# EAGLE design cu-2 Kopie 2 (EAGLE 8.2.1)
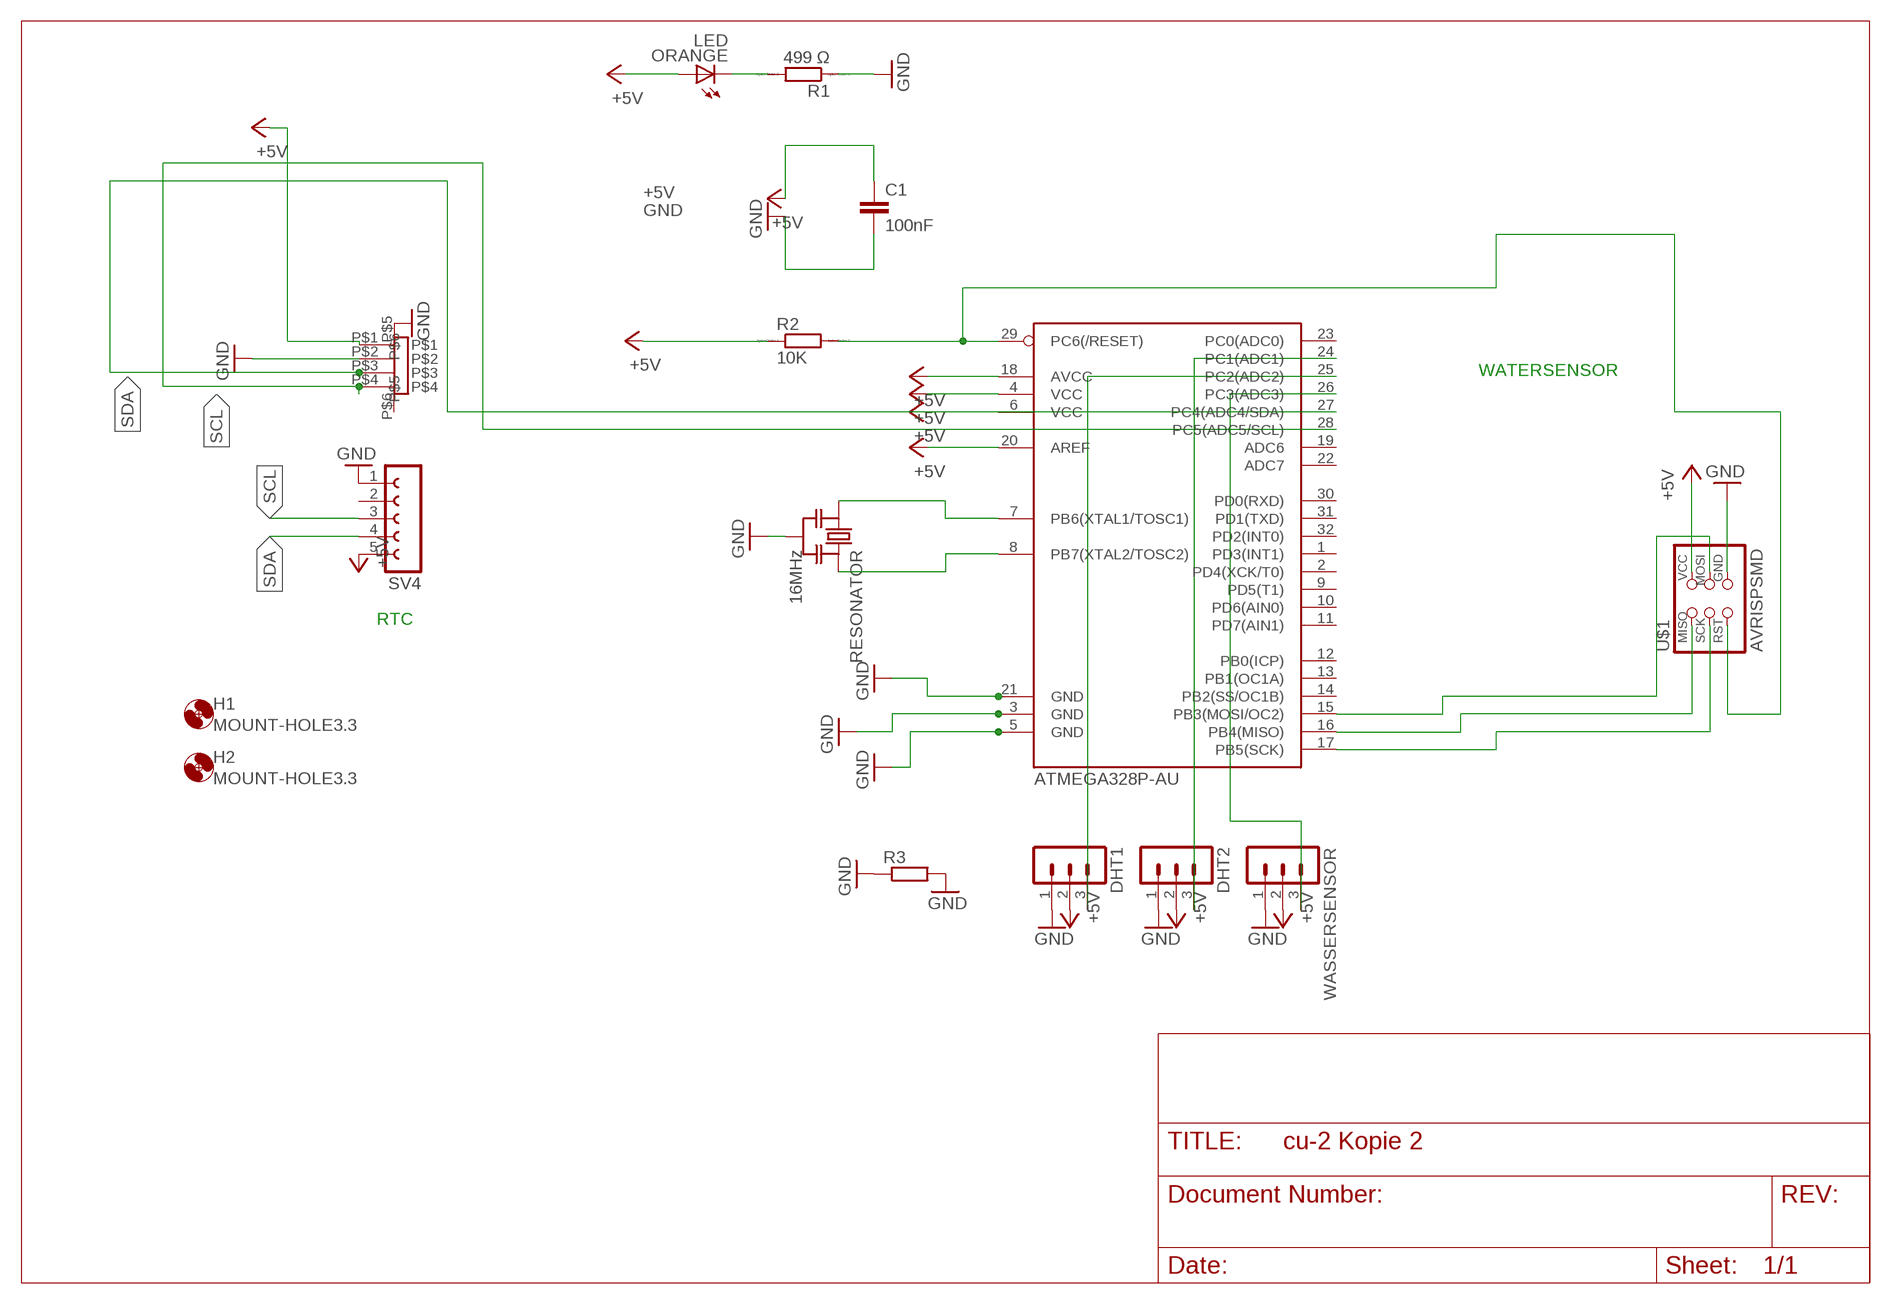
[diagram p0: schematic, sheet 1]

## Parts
ATMEGA328P-AU  ATMEGA88-THIN  [TQFP32-08THIN]
C1  100nF  C-EUC1206  [C1206]
DHT1  MA03-1  [MA03-1]
DHT2  MA03-1  [MA03-1]
H1  MOUNT-HOLE3.3  [3,3]
H2  MOUNT-HOLE3.3  [3,3]
ORANGE  LED  [LED1206]
R1  499 Ω  RR1206  [R1206]
R2  10K  RR1206  [R1206]
R3  R-EU_0207/10  [0207/10]
RESONATOR  16MHz  RESONATOR-MURATACSTCR_G  [RESONATOR_MURATA3]
SV4  FE05-1  [FE05-1]
U$1  AVRISPSMD  [2X03SMD]
U$2  PHP4_SM4  [PH4P_SM4]
WASSERSENSOR  MA03-1  [MA03-1]

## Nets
+5V: ATMEGA328P-AU.4(VCC) ATMEGA328P-AU.6(VCC) ATMEGA328P-AU.18(AVCC) ATMEGA328P-AU.20(AREF) C1.1 DHT1.2 DHT2.2 ORANGE.1(A) R2.1 SV4.5 U$1.2(VCC) U$2.P$1 WASSERSENSOR.2
GND: ATMEGA328P-AU.3(GND) ATMEGA328P-AU.5(GND) ATMEGA328P-AU.21(GND) C1.2 DHT1.1 DHT2.1 R1.1 R3.1 R3.2 RESONATOR.2 SV4.1 U$1.6(GND) U$2.P$2 U$2.P$5 WASSERSENSOR.1
N$2: ATMEGA328P-AU.26(PC3(ADC3)) WASSERSENSOR.3
N$3: ATMEGA328P-AU.24(PC1(ADC1)) DHT2.3
N$4: ATMEGA328P-AU.25(PC2(ADC2)) DHT1.3
N$6: ATMEGA328P-AU.15(PB3(MOSI/OC2)) U$1.4(MOSI)
N$19: ATMEGA328P-AU.17(PB5(SCK)) U$1.3(SCK)
N$20: ATMEGA328P-AU.16(PB4(MISO)) U$1.1(MISO)
N$24: ORANGE.2(C) R1.2
N$27: ATMEGA328P-AU.7(PB6(XTAL1/TOSC1)) RESONATOR.1
N$28: ATMEGA328P-AU.8(PB7(XTAL2/TOSC2)) RESONATOR.3
N$29: ATMEGA328P-AU.29(PC6(/RESET)) R2.2 U$1.5(RST)
SCL: ATMEGA328P-AU.28(PC5(ADC5/SCL)) SV4.3 U$2.P$4
SDA: ATMEGA328P-AU.27(PC4(ADC4/SDA)) SV4.4 U$2.P$3
Unconnected: ATMEGA328P-AU.1(PD3(INT1)) ATMEGA328P-AU.2(PD4(XCK/T0)) ATMEGA328P-AU.9(PD5(T1)) ATMEGA328P-AU.10(PD6(AIN0)) ATMEGA328P-AU.11(PD7(AIN1)) ATMEGA328P-AU.12(PB0(ICP)) ATMEGA328P-AU.13(PB1(OC1A)) ATMEGA328P-AU.14(PB2(SS/OC1B)) ATMEGA328P-AU.19(ADC6) ATMEGA328P-AU.22(ADC7) ATMEGA328P-AU.23(PC0(ADC0)) ATMEGA328P-AU.30(PD0(RXD)) ATMEGA328P-AU.31(PD1(TXD)) ATMEGA328P-AU.32(PD2(INT0)) SV4.2 U$2.P$6

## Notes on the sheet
- WATERSENSOR
- RTC

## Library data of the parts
ATMEGA328P-AU = fab:ATMEGA88-THIN
C1 = rcl:C-EU: CAPACITOR, European symbol
DHT1 DHT2 WASSERSENSOR = con-lstb:MA03-1: PIN HEADER; OC_FARNELL: unknown; OC_NEWARK: unknown
H1 H2 = holes:MOUNT-HOLE: MOUNTING HOLE with drill center marker
ORANGE = fab:LED: LED
R1 R2 = eagle-ltspice:R: RESISTOR, European symbol; SPICEMODEL: NONE; SPICEPREFIX: R
R3 = rcl:R-EU_: RESISTOR, European symbol
RESONATOR = m-pad-2.1:RESONATOR-MURATA: Murata ceramic Resonator "ceralock" CSTCE series with built in load capacitance +- 0.5% tolerance 12.51MHz to 19.99MHz 16MHz murata part#: CSTCE16M0V53-R0 16MHz digikey part#: 490-1198-1-ND $1.33 each
SV4 = con-lsta:FE05-1: FEMALE HEADER; OC_FARNELL: unknown; OC_NEWARK: unknown
U$1 = fab:AVRISP
U$2 = jst_ph_topo:PHP4_SM4

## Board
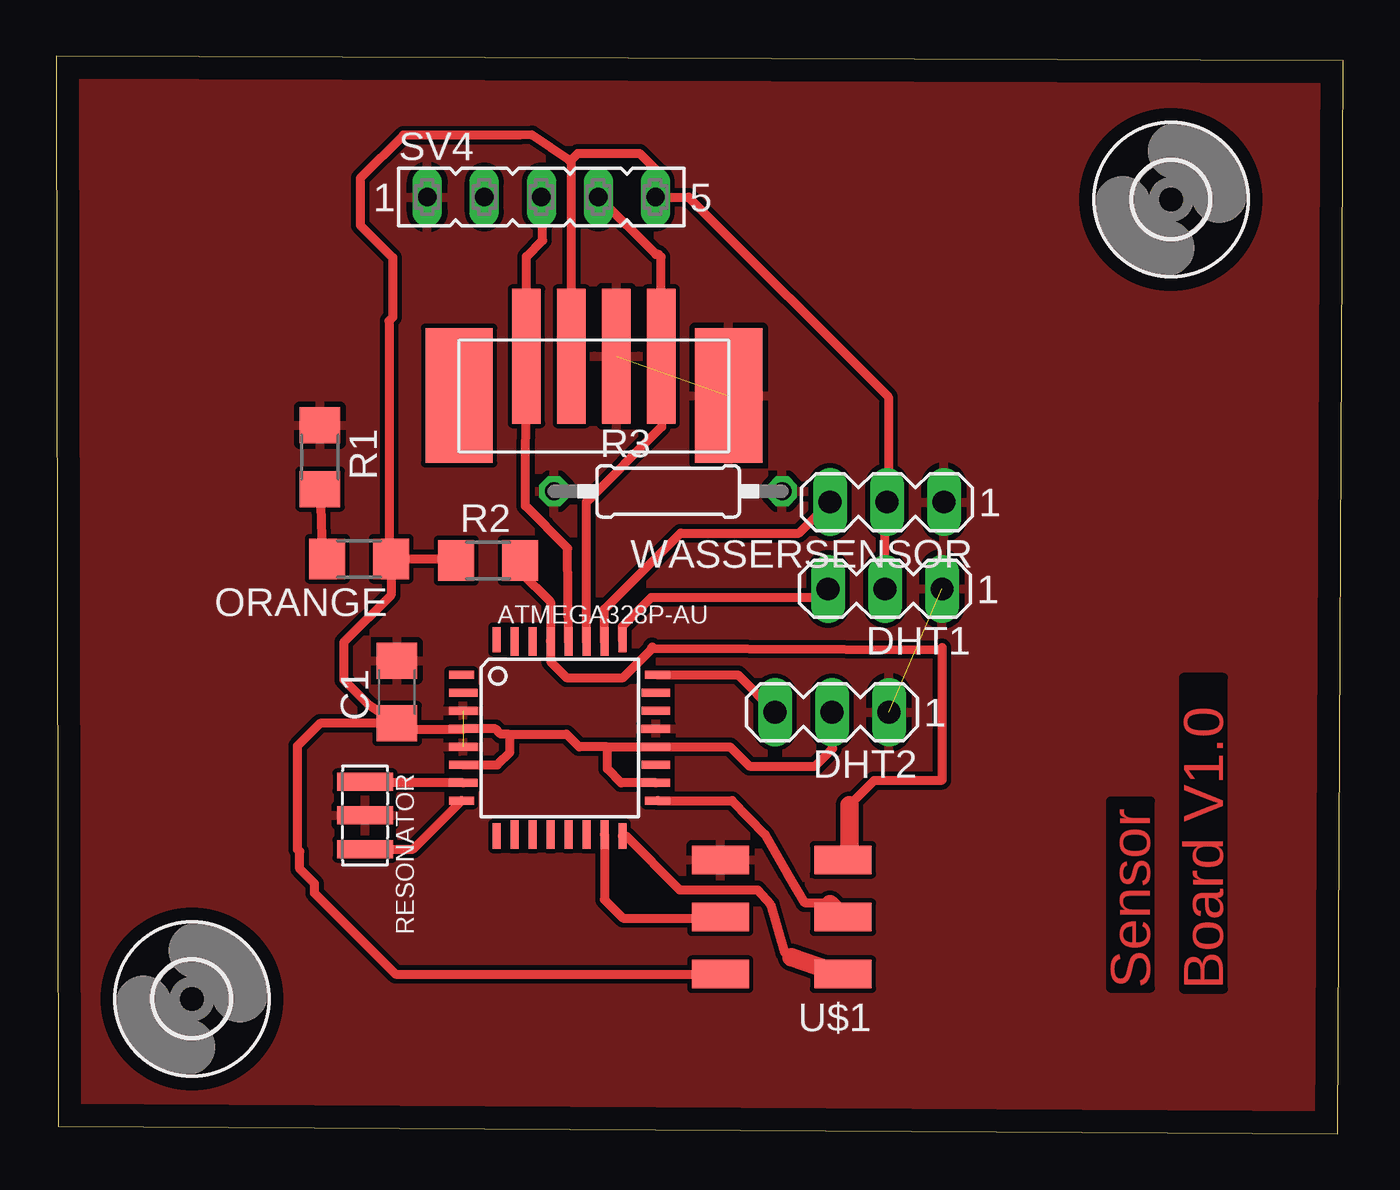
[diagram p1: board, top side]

Size 57.31 x 47.95 mm. Coordinates in mm from the lower left corner, seen from the top.
Outline: 0.09,0.32 57.06,0 57.31,47.75 0,47.95 0.09,0.32
Copper layers (1*16): Top 0.035mm / dielectric 1.5mm / Bottom 0.035mm
Design rules "default": minimum track width 10mil, minimum drill 24mil, track to track 8mil, track to pad 8mil, pad to pad 8mil, via to via 8mil, smd to smd 8mil, copper to edge 40mil, drill to drill 8mil, minimum pad ring 10mil, minimum via ring 8mil, stop-mask expansion 4mil, vias tented up to drill 0mil, thermal gap 10mil

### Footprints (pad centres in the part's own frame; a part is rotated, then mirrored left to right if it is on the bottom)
TQFP32-08THIN = smd 1.118 x 0.356: 1 -4.369,2.8; 8 -4.369,-2.8; 17 4.369,-2.8; 24 4.369,2.8 | smd 1.27 x 0.356: 2 -4.293,2; 3 -4.293,1.2; 4 -4.293,0.4; 5 -4.293,-0.4; 6 -4.293,-1.2; 7 -4.293,-2; 18 4.293,-2; 19 4.293,-1.2; 20 4.293,-0.4; 21 4.293,0.4; 22 4.293,1.2; 23 4.293,2 | smd 0.356 x 1.118: 9 -2.8,-4.369; 16 2.8,-4.369; 25 2.8,4.369; 32 -2.8,4.369 | smd 0.356 x 1.27: 10 -2,-4.293; 14 1.2,-4.293; 15 2,-4.293; 26 2,4.293; 27 1.2,4.293; 31 -2,4.293 | smd 0.35 x 1.27: 11 -1.2,-4.293; 12 -0.4,-4.293; 13 0.4,-4.293; 28 0.4,4.293; 29 -0.4,4.293; 30 -1.2,4.293
C1206 = smd 1.6 x 1.8: 1 -1.4,0; 2 1.4,0
MA03-1 = drill 1.016 long: 1 -2.54,0; 2 0,0; 3 2.54,0
3,3 = hole 3.3: 0,0
LED1206 = smd 1.6 x 1.803: 1 -1.422,0; 2 1.422,0
R1206 = smd 1.6 x 1.803: 1 -1.422,0; 2 1.422,0
0207/10 = drill 0.813 octagon: 1 -5.08,0; 2 5.08,0
RESONATOR_MURATA3 = smd 0.8 x 2.5: 1 -1.5,0; 2 0,0; 3 1.5,0
FE05-1 = drill 0.813 long: 1 -5.08,0; 2 -2.54,0; 3 0,0; 4 2.54,0; 5 5.08,0
2X03SMD = smd 2.54 x 1.27: 1 -2.54,2.54; 2 2.92,2.54; 3 -2.54,0; 4 2.92,0; 5 -2.54,-2.54; 6 2.92,-2.54
PH4P_SM4 = smd 6 x 1.27: P$1 2,2; P$2 2,4; P$3 2,6; P$4 2,0 | smd 6 x 3: P$5 3.75,9; P$6 3.75,-3

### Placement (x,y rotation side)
ATMEGA328P-AU  22.41,17.61 0 top
C1  15.18,19.65 90 top
DHT1  36.91,24.24 180 top
DHT2  34.55,18.76 180 top
H1  49.63,41.57 0 top
H2  6.04,6 0 top
ORANGE  13.49,25.58 180 top
R1  11.75,30.11 270 top
R2  19.24,25.51 0 top
R3  27.25,28.59 0 top
RESONATOR  13.75,14.16 270 top
SV4  21.6,41.68 0 top
U$1  32.49,9.64 180 top
U$2  20.94,36.6 270 top
WASSERSENSOR  36.99,28.11 180 top

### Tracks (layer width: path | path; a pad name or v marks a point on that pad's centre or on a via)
+5V
  Top 0.406: 24.53,17.21 ATMEGA328P-AU.20 30,17.21 30.86,16.35 33.79,16.35 34.57,17.13 34.57,18.73 DHT2.2 | 24.53,17.21 23.28,17.21 22.72,17.77 20.11,17.77 | 20.11,17.77 19.8,17.77 19.56,18.01 ATMEGA328P-AU.4 18.1,18 17.05,18 15.92,18 C1.1 | ATMEGA328P-AU.18 25.16,15.61 24.55,16.23 24.55,17.2 24.53,17.21 | ATMEGA328P-AU.6 19.64,16.41 20.2,16.97 20.2,17.68 20.11,17.77 | C1.1 13.91,19.09 12.81,20.19 12.81,21.86 14.91,23.96 ORANGE.1 | U$1.2 15.11,7.1 11.51,10.7 11.51,11.12 10.85,11.78 10.85,12.55 10.75,12.65 10.75,17.25 11.75,18.25 C1.1 | ORANGE.1 14.81,25.68 14.81,36.17 14.98,36.34 14.98,38.99 13.54,40.44 13.54,42.51 15.46,44.44 20.65,44.44 21.19,44.45 22.83,43.34 22.94,43.34 | ORANGE.1 17.74,25.58 R2.1 | DHT1.2 36.91,28.02 WASSERSENSOR.2 37.05,28.17 37.05,32.79 28.16,41.68 SV4.5 26.76,41.76 26.76,42.85 25.97,43.63 23.24,43.63 22.94,43.34 | U$2.P$1 22.94,43.34
GND  (3 unrouted)
  pour Top: 60.78,49.62 -2.43,49.71 -2.14,-2.99 61.33,-2.93
N$2
  Top 0.406: ATMEGA328P-AU.26 24.41,23.34 27.8,26.72 33.07,26.72 WASSERSENSOR.3
N$3
  Top 0.406: ATMEGA328P-AU.24 30.35,20.41 DHT2.3
N$4
  Top 0.406: ATMEGA328P-AU.25 25.21,22.57 26.51,23.87 33.99,23.87 DHT1.3
N$6
  Top 0.406: ATMEGA328P-AU.15 24.41,10.41 25.24,9.58 29.52,9.58 U$1.4
N$19
  Top 0.406: ATMEGA328P-AU.17 30.09,14.81 31.56,13.3 32.55,11.6 32.96,10.87 33.33,10.28 34.39,10.28 34.45,10.21
  Top 0.813: 34.45,10.21 U$1.3
N$20
  Top 0.406: ATMEGA328P-AU.16 25.36,13.25 27.76,10.84 31.23,10.84 31.79,10.2 32.43,8.06 32.74,7.85 | 35,7.06 U$1.1
  Top 0.813: 32.74,7.85 35,7.06
N$24
  Top 0.406: R1.2 11.84,25.81 ORANGE.2
N$27
  Top 0.406: ATMEGA328P-AU.7 13.8,15.61 RESONATOR.1
N$28
  Top 0.406: RESONATOR.3 15.89,12.66 ATMEGA328P-AU.8
N$29
  Top 0.406: 35.32,12.47 U$1.5 | R2.2 20.66,25.02 22.01,23.67 ATMEGA328P-AU.29 22.01,21 22.72,20.29 25.24,20.29 26.5,21.55 26.54,21.67 26.53,21.61 39.43,21.54 39.45,21.63 39.45,15.73 39.36,15.71 36.41,15.71 35.32,14.62
  Top 0.813: 35.32,14.62 35.32,12.47
SCL
  Top 0.406: ATMEGA328P-AU.28 22.77,26.05 20.89,27.93 20.93,33.85 20.82,33.96 20.82,34.48 U$2.P$4 20.94,39.04 21.66,39.75 21.66,41.63 SV4.3
SDA
  Top 0.406: ATMEGA328P-AU.27 23.61,28.11 26.96,31.45 26.96,34.58 U$2.P$3 26.94,39.01 26.82,39.13 26.7,39.13 SV4.4

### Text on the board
Top: Sensor | Board V1.0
